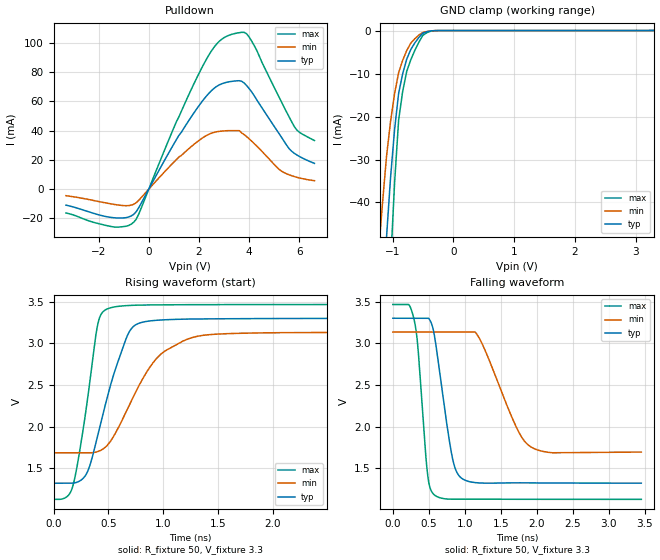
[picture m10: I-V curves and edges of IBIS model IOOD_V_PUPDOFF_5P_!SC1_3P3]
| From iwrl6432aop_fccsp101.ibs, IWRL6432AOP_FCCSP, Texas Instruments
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|   Model Cell IOOD_V_PUPDOFF_5P_!SC1_3P3
|IOOD_V_PUPDOFF_5P_!SC1_3P3
[Model]   IOOD_V_PUPDOFF_5P_!SC1_3P3
Model_type   I/O_open_drain
Polarity   Non-Inverting
Enable   Active-Low
Vinl =  0.8V
Vinh =  2V
Cref =  15pF
Rref =  100.0000M
Vref =  0V
Vmeas =  1.65
|   typ   min   max
C_comp   2.059994p   1.862014p   2.067327p
[Model Spec]
Vinl   0.8V   0.8V   0.8V
Vinh   2V   2V   2V
[Temperature Range]   25   125   -40
[Voltage Range]   3.3   3.135   3.465
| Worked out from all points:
|   slope of the pulldown table from 0 to 0.495 V, typ, clamps not added: 31.8 ohm
|   GND clamp passes 1 mA (typ) near -0.53 V on its own axis
|   rising waveform, R_fixture 50, V_fixture 3.3: 20-80 % time 251ps typ, 371ps min, 151ps max; typ from 1.32 V to 3.3 V
|   falling waveform, R_fixture 50, V_fixture 3.3: 20-80 % time 196ps typ, 407ps min, 120ps max; typ from 3.3 V to 1.32 V
| Where Nom  PVT is Nominal Process, 3.3V, 25C
|   Fast PVT is Strong Process,  3.465V, -40C
|   Slow PVT is Weak Process,   3.135V, 125C
[Pulldown]
|   voltage   I(typ)   I(min)   I(max)
-3.3V     -10.92mA   -4.469mA   -16.24mA
-1.4V     -19.52mA   -10.37mA   -25.81mA
-600mV    -17.22mA   -10.34mA   -22.6mA
-400mV    -12.67mA   -7.623mA   -17.05mA
1.2V      36.7mA     21.92mA    49.35mA
2.1V      59.3mA     34.49mA    82.4mA
2.7V      70.09mA    39.15mA    99.03mA
3.3V      73.56mA    39.95mA    105.7mA
3.9V      70.66mA    35.84mA    106mA
5.2V      37.64mA    13.39mA    62.46mA
5.8V      24.43mA    8.578mA    42.66mA
6.6V      17.6mA     5.765mA    33.17mA
[GND_clamp]
|   voltage   I(typ)   I(min)   I(max)
-3.3V     -787.2mA   -627.7mA   -1.235A
-1.233V   -85.66mA   -52.14mA   -138.8mA
-1.167V   -66.47mA   -40.37mA   -107.7mA
-1.1V     -48.25mA   -29.37mA   -77.98mA
-1.033V   -34.27mA   -21.19mA   -54.56mA
-966.7mV  -23.06mA   -14.66mA   -35.5mA
-900mV    -14.61mA   -9.789mA   -20.83mA
-833.3mV  -10.05mA   -6.934mA   -14.15mA
-700mV    -4.416mA   -2.931mA   -6.81mA
-500mV    -621.6uA   -443.6uA   -1.094mA
-300mV    -17.13uA   -24.35uA   -23.51uA
3.3V      4.589uA    5.188uA    6.318uA
[Ramp]
| variable   typ   min   max
dV/dt_f  1.1959432/0.19778326n 0.88997478/0.42010629n  1.4076426/0.12045204n
dV/dt_r  1.1917501/0.23458044n 0.88925157/0.46804062n  1.4206668/0.14157829n
R_load = 50
[Rising Waveform]
R_fixture = 50
V_fixture = 3.3
V_fixture_min = 3.135
V_fixture_max = 3.465
|   time   V(typ)   V(min)   V(max)
0s        1.323V     1.687V     1.129V
178.2ps   1.324V     1.687V     1.297V
304.7ps   1.446V     1.687V     2.276V
398.7ps   1.871V     1.7V       3.195V
481.7ps   2.309V     1.765V     3.406V
653.8ps   3.025V     2.155V     3.45V
722.6ps   3.193V     2.343V     3.455V
946.6ps   3.276V     2.827V     3.46V
1.239ns   3.29V      3.057V     3.463V
3.453ns   3.299V     3.131V     3.465V
[Falling Waveform]
R_fixture = 50
V_fixture = 3.3
V_fixture_min = 3.135
V_fixture_max = 3.465
|   time   V(typ)   V(min)   V(max)
0s        3.299V     3.134V     3.464V
297.1ps   3.299V     3.134V     3.277V
347.5ps   3.299V     3.134V     2.96V
479.2ps   3.299V     3.134V     1.457V
581.1ps   3.075V     3.134V     1.179V
822.1ps   1.65V      3.134V     1.13V
962ps     1.378V     3.134V     1.13V
1.186ns   1.326V     3.084V     1.13V
1.91ns    1.326V     1.762V     1.129V
3.453ns   1.322V     1.695V     1.129V
